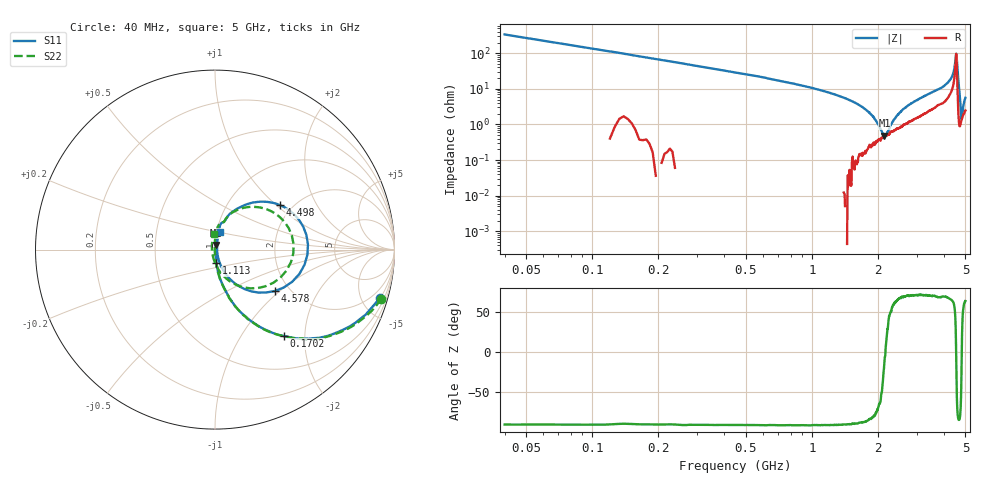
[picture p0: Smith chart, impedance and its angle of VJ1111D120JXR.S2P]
! VJ1111D120JXR
! DATE 02/16/2022  09:57
! CAPACITORS MOUNTED IN SERIES ON 25 MIL THICK MICROSTRIP SUBSTRATE
# GHz  S  MA  R  50.00
!  FREQ  S11M  S11A  S21M  S21A  S12M  S12A  S22M  S22A
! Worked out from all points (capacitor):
!   801 points, 40 MHz to 5 GHz, reference 50 ohm
!   read as one part in series: C = 11.8 pF near 64.8 MHz
!   lowest |Z| = 480 mohm at 2.142 GHz (marker M1)
!   series resonance near 2.163 GHz, so ESL is about 460 pH
!   S11 on the Smith chart (normalised r, x): 40 MHz: 1.05, -6.72; 170.2 MHz: 1.01, -1.57; 1.113 GHz: 1.00, -0.15; 4.498 GHz: 1.73, +1.06; 4.578 GHz: 1.68, -0.93; 5 GHz: 1.03, +0.20
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0.04  0.9567 -16.5  0.2855 73.5  0.2847 73.5  0.9659 -16.5
0.1702  0.6147 -51.6  0.7839 38.4  0.7842 38.8  0.6175 -51.4
0.381  0.3197 -71.0  0.9484 19.3  0.9528 19.1  0.3233 -71.1
0.8708  0.1181 -82.2  0.9934 8.1  0.9971 7.9  0.1183 -82.8
1.1126  0.07588 -83.8  0.9958 5.9  1 5.9  0.07538 -85.8
1.466  0.03171 -83.6  0.9961 4.0  1.001 3.8  0.03187 -89.3
1.6954  0.009802 -71.3  0.9944 3.1  1 2.9  0.01016 -95.6
1.745  0.005788 -59.1  0.9944 2.9  1 2.7  0.006105 -101.6
1.8132  0.003249 19.7  0.9938 2.7  0.9987 2.5  0.001066 -175.4
1.9248  0.01031 70.4  0.9931 2.3  0.9979 2.1  0.00889 100.2
2.1418  0.02672 80.8  0.9903 1.7  0.9953 1.5  0.02473 91.8
2.52  0.05124 81.7  0.9839 0.7  0.9889 0.5  0.0493 90.5
3.3508  0.1045 79.2  0.9622 -1.4  0.967 -1.5  0.09524 84.4
4.1754  0.1952 69.4  0.9196 -5.0  0.9228 -5.0  0.1608 72.4
4.3986  0.2916 57.2  0.8504 -9.0  0.854 -8.9  0.2384 63.2
4.4978  0.4392 34.3  0.6637 -12.4  0.6669 -12.5  0.3678 37.3
4.5412  0.5187 3.2  0.5004 6.8  0.5029 6.8  0.4385 4.2
4.5784  0.4056 -34.7  0.7324 24.9  0.7364 24.7  0.3472 -36.1
4.6342  0.1599 -65.3  0.9468 14.1  0.9513 14.0  0.1399 -74.6
4.7334  0.01167 14.5  0.9768 5.3  0.9807 5.2  0.01705 -172.4
4.8326  0.05897 75.9  0.9687 2.2  0.9723 2.2  0.05052 106.8
5  0.1016 75.6  0.9554 -0.1  0.9605 -0.2  0.08796 92.9
